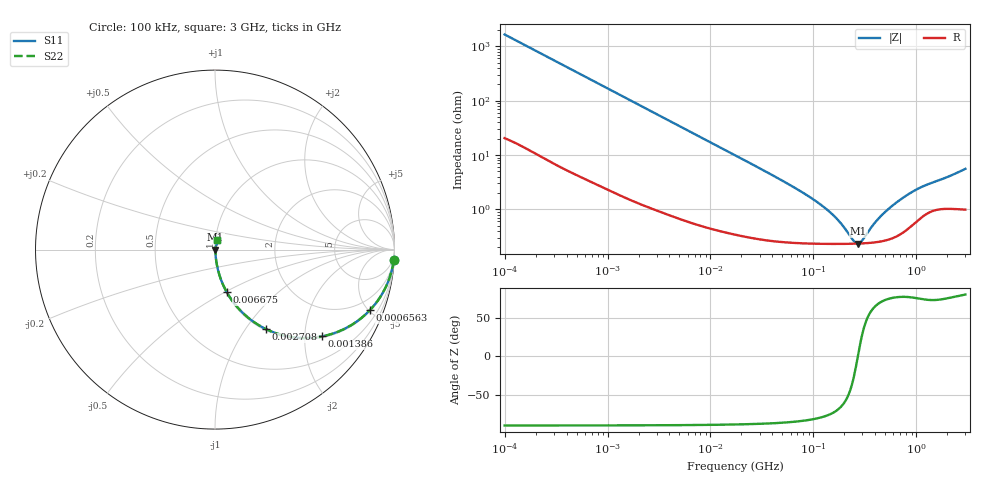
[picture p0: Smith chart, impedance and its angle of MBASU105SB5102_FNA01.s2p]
! MBASU105SB5102_FNA01  S-PARAMETER MODEL  ( Standard Model )
! Model Generated by TAIYO YUDEN Corporation (http://www.ty-top.com)
! Version 1.0
! TAIYO YUDEN Control No. 220601
! Copyright(c) 2013 TAIYO YUDEN CO.,LTD. All Rights Reserved.
! Product Description (link to TY-COMPAS)
! https://ds.yuden.co.jp/TYCOMPAS/or/detail?pn=MBASU105SB5102KFNA01&u=M
! Products Name : Multilayer Ceramic Capacitors
! Characteristics :
!  Capacitance : 1000 [pF] , Rated Voltage : 50 [V] , TCC : X5R
!  Case Size : 1.0 x 0.5 / 0.039 x 0.02 [mm/inch] , Thickness : 0.5 / 0.02 [mm/inch]
!  (Conditions: Temperature = 25 [degC] , DC Bias Voltage = 0 [V])
! External Node Assignments :
!  1  o---| |---o  2
! GND o---------o GND
! Frequency Range : 100kHz  -  3GHz  [ 401 STEP ]
# MHZ S RI R 50
! Freq[MHz].  S11 Real  S11 Imag  S21 Real  S21 Imag  S12 Real  S12 Imag  S22 Real  S22 Imag
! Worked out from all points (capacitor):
!   401 points, 100 kHz to 3 GHz, reference 50 ohm
!   read as one part in series: C = 959 pF near 105.3 kHz
!   lowest |Z| = 235 mohm at 273 MHz (marker M1)
!   series resonance near 270.6 MHz, so ESL is about 360 pH
!   S11 on the Smith chart (normalised r, x): 100 kHz: 1, -33; 656.3 kHz: 1.07, -5.12; 1.386 MHz: 1.03, -2.44; 2.708 MHz: 1.02, -1.26; 6.675 MHz: 1.01, -0.51; 3 GHz: 1.02, +0.11
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0.1  0.9956 -0.0601  0.00438 0.0601  0.00438 0.0601  0.9956 -0.0601
0.246461  0.9769 -0.144  0.0231 0.144  0.0231 0.144  0.9769 -0.144
0.562235  0.8961 -0.2988  0.1039 0.2988  0.1039 0.2988  0.8961 -0.2988
0.656258  0.8645 -0.3358  0.1355 0.3358  0.1355 0.3358  0.8645 -0.3358
0.941399  0.7593 -0.4208  0.2407 0.4208  0.2407 0.4208  0.7593 -0.4208
1.385689  0.5969 -0.4835  0.4031 0.4835  0.4031 0.4835  0.5969 -0.4835
1.937191  0.4347 -0.4882  0.5653 0.4882  0.5653 0.4882  0.4347 -0.4882
2.708188  0.2858 -0.4437  0.7142 0.4437  0.7142 0.4437  0.2858 -0.4437
3.161081  0.2286 -0.4115  0.7714 0.4115  0.7714 0.4115  0.2286 -0.4115
6.674626  0.0663 -0.2382  0.9337 0.2382  0.9337 0.2382  0.0663 -0.2382
17.7727  0.0126 -0.0953  0.9874 0.0953  0.9874 0.0953  0.0126 -0.0953
51.12795  0.00355 -0.0326  0.9964 0.0326  0.9964 0.0326  0.00355 -0.0326
97.38194  0.00258 -0.0155  0.9974 0.0155  0.9974 0.0155  0.00258 -0.0155
154.8634  0.00237 -0.00756  0.9976 0.00756  0.9976 0.00756  0.00237 -0.00756
190.323  0.00233 -0.00463  0.9977 0.00463  0.9977 0.00463  0.00233 -0.00463
246.2744  0.00233 -0.00122  0.9977 0.00122  0.9977 0.00122  0.00233 -0.00122
273.0175  0.00234 0.000115  0.9977 -0.000115  0.9977 -0.000115  0.00234 0.000115
302.6647  0.00237 0.00146  0.9976 -0.00146  0.9976 -0.00146  0.00237 0.00146
423.1245  0.00254 0.00604  0.9975 -0.00604  0.9975 -0.00604  0.00254 0.00604
547.5153  0.0029 0.0101  0.9971 -0.0101  0.9971 -0.0101  0.0029 0.0101
1042.837  0.00681 0.023  0.9932 -0.023  0.9932 -0.023  0.00681 0.023
3000  0.0127 0.0536  0.9873 -0.0536  0.9873 -0.0536  0.0127 0.0536
